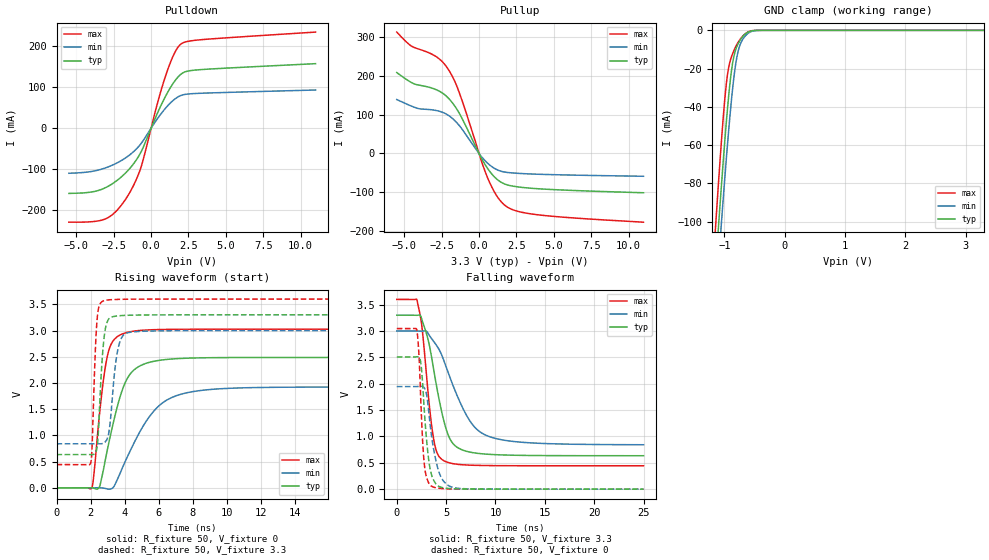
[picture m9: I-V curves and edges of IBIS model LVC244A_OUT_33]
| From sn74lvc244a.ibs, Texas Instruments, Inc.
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[Model]   LVC244A_OUT_33
Model_type  3-state
Enable   Active-Low
Vref =   0
Rref =   500
Cref =   50p
Vmeas =   1.5
| variable   typ   min   max
C_comp   3.70pF   3.32pF   4.27pF
| C_pullup   8.34pF   3.87pF   12.57pF
| C_pulldown   6.60pF   3.56pF   12.66pF
| C_tri-state   3.70pF   3.32pF   4.27pF
[Temperature Range]   40   100   -40
| Ambient temperature   25   85   -40
[Voltage range]   3.3   3   3.6
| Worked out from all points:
|   slope of the pulldown table from 0 to 0.495 V, typ, clamps not added: 11.7 ohm
|   slope of the pullup table from 0 to 0.495 V, typ, clamps not added: 14.4 ohm
|   GND clamp passes 1 mA (typ) near -0.61 V on its own axis
|   rising waveform, R_fixture 50, V_fixture 0: 20-80 % time 1.16ns typ, 2.06ns min, 628ps max; typ from 0 V to 2.49 V
|   falling waveform, R_fixture 50, V_fixture 3.3: 20-80 % time 1.7ns typ, 2.99ns min, 1.02ns max; typ from 3.3 V to 0.634 V
|   rising waveform, R_fixture 50, V_fixture 3.3: 20-80 % time 285ps typ, 402ps min, 212ps max; typ from 0.634 V to 3.3 V
|   falling waveform, R_fixture 50, V_fixture 0: 20-80 % time 660ps typ, 977ps min, 449ps max; typ from 2.51 V to 0 V
[GND Clamp]
| LVC244A_OUT_33
|   Voltage   I(typ)   I(min)   I(max)
-5.5V     -2.404A    -2.35A     -2.478A
-1.16V    -130.8mA   -149.3mA   -109mA
-1.135V   -119.3mA   -138.1mA   -96.92mA
-1.095V   -101.1mA   -120.3mA   -78.15mA
-1.065V   -87.8mA    -107.3mA   -64.63mA
-1.05V    -81.28mA   -100.8mA   -58.11mA
-960mV    -44.92mA   -63.9mA    -25.79mA
-905mV    -26.86mA   -43.63mA   -16.07mA
-860mV    -16.39mA   -29.29mA   -11.91mA
-760mV    -6.281mA   -9.433mA   -5.644mA
-610mV    -992.5uA   -1.611mA   -858.5uA
3.3V      99.71pA    617.3nA    40.99pA
[Pulldown]
| LVC244A_OUT_33
|   Voltage   I(typ)   I(min)   I(max)
-5.5V     -158.7mA   -109.7mA   -228.6mA
-3.025V   -144.3mA   -96.32mA   -220.3mA
-2.33V    -128.6mA   -85.51mA   -201.7mA
-1.6V     -105mA     -69.54mA   -167mA
-1.08V    -82mA      -53.93mA   -132.1mA
-665mV    -57.29mA   -37.15mA   -93.9mA
450mV     38.69mA    24.45mA    63.98mA
1.09V     86mA       53.75mA    140.1mA
1.585V    114.8mA    70.7mA     184mA
1.99V     131.2mA    79.41mA    204.4mA
3.175V    142.1mA    84.7mA     214.6mA
11V       156.9mA    92.85mA    233.8mA
[Pullup]
| LVC244A_OUT_33
|   Voltage   I(typ)   I(min)   I(max)
-5.5V     208.9mA    139.3mA    313.5mA
-4.515V   183.1mA    122.2mA    277.2mA
-2.765V   163mA      110.1mA    247.3mA
-2.02V    141.7mA    97.67mA    215.1mA
-1.29V    101.8mA    70.66mA    153.7mA
170mV     -12.86mA   -8.44mA    -20.6mA
585mV     -39.44mA   -25.5mA    -63.88mA
1.17V     -65.66mA   -41.32mA   -108.5mA
1.765V    -79.61mA   -48.34mA   -135mA
2.54V     -86.1mA    -51.21mA   -148.9mA
3.93V     -91.11mA   -53.65mA   -158.4mA
11V       -101.5mA   -58.93mA   -177.6mA
[Ramp]
| LVC244A_OUT_33
| variable   typ   min   max
dV/dt_r   1.51/1.17E-09   1.17/2.07E-09   1.83/6.32E-10
dV/dt_f   1.60/1.70E-09   1.30/2.99E-09   1.90/1.02E-09
R_load = 50
[Rising Waveform]
| LVC244A_OUT_33
R_fixture =   50
C_fixture =   0
L_fixture =   0
V_fixture =   0
V_fixture_min = 0
V_fixture_max = 0
|   Time   V(typ)   V(min)   V(max)
0s        392.8pV    3.681nV    162.3pV
2.085ns   -103.4uV   311.3uV    13.92mV
2.52ns    18.47mV    1.313mV    1.4V
2.95ns    675.6mV    -19.04mV   2.464V
3.29ns    1.183V     -3.49mV    2.789V
3.905ns   1.908V     412.3mV    2.941V
4.555ns   2.252V     861.9mV    2.989V
5.69ns    2.412V     1.457V     3.016V
7.63ns    2.472V     1.812V     3.024V
24.99ns   2.486V     1.923V     3.025V
[Falling Waveform]
| LVC244A_OUT_33
R_fixture =   50
C_fixture =   0
L_fixture =   0
V_fixture =   3.3
V_fixture_min = 3
V_fixture_max = 3.6
|   Time   V(typ)   V(min)   V(max)
0s        3.3V       3V         3.6V
2.045ns   3.298V     3V         3.59V
2.55ns    3.211V     2.999V     3.076V
3.69ns    2.323V     2.815V     1.001V
4.075ns   1.91V      2.713V     692.2mV
4.65ns    1.387V     2.498V     553.7mV
5.91ns    824.2mV    1.868V     477.5mV
7.52ns    698.9mV    1.264V     454.9mV
9.085ns   664.2mV    1.019V     448.3mV
24.99ns   634.4mV    842.4mV    443.6mV
[Rising Waveform]
| LVC244A_OUT_33
R_fixture =   50
C_fixture =   0
L_fixture =   0
V_fixture =   3.3
V_fixture_min = 3
V_fixture_max = 3.6
|   Time   V(typ)   V(min)   V(max)
0s        634.3mV    840.5mV    443.6mV
2ns       634.8mV    840.7mV    470.4mV
2.085ns   634.7mV    840.7mV    782.7mV
2.255ns   653.2mV    840.7mV    2.439V
2.37ns    755.2mV    840.5mV    3.172V
2.77ns    2.806V     855.5mV    3.568V
3.085ns   3.228V     1.086V     3.585V
3.6ns     3.279V     2.641V     3.594V
4.12ns    3.29V      2.952V     3.597V
24.99ns   3.3V       3V         3.6V
[Falling Waveform]
| LVC244A_OUT_33
R_fixture =   50
C_fixture =   0
L_fixture =   0
V_fixture =   0
V_fixture_min = 0
V_fixture_max = 0
|   Time   V(typ)   V(min)   V(max)
0s        2.509V     1.946V     3.047V
2.025ns   2.51V      1.946V     3.026V
2.24ns    2.504V     1.948V     2.572V
2.43ns    2.4V       1.952V     1.697V
2.765ns   1.561V     1.927V     522.3mV
3.135ns   717.3mV    1.645V     161.3mV
3.495ns   289.9mV    1.044V     59.28mV
4.37ns    43.82mV    275.9mV    15.76mV
5.69ns    7.801mV    32.31mV    2.842mV
24.99ns   38.57uV    93.03uV    16.2uV
